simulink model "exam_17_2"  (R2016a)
settings: Solver=ode15s  StartTime=0.0  StopTime=0.2  RelTol=1e-3
libraries: powerlib x9

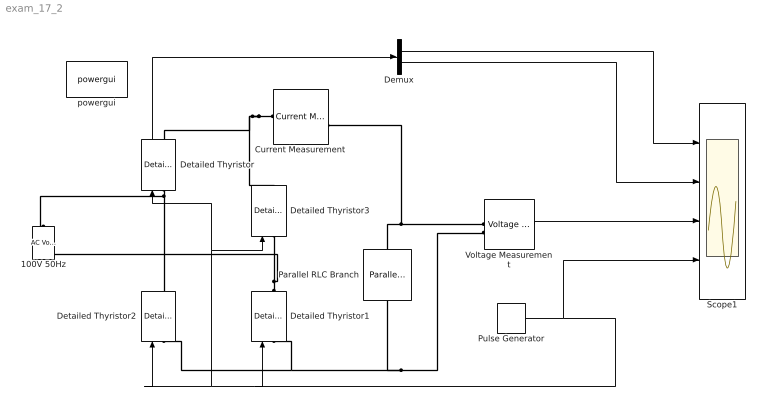
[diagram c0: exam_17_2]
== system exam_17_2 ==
  100V 50Hz : powerlib/Electrical Sources/AC Voltage Source  Amplitude=100  Phase=0  Frequency=50  SampleTime=0  Measurements=None  BusType=swing  Pref=10e3  Qref=0  Qmin=-inf  Qmax=+inf
  Current Measurement : powerlib/Measurements/Current Measurement  PhasorSimulation=off  OutputType=Complex  PSBequivalent=0
  Demux : Demux  Outputs=2
  Detailed Thyristor{,1..3} (4 alike) : powerlib/Power Electronics/Detailed Thyristor  Ron=0.001  Lon=1e-3  Vf=0.8  IL=0.1  Tq=100e-6  IC=0  Rs=500  Cs=250e-9  Measurements=on
  Parallel RLC Branch : powerlib/Elements/Parallel RLC Branch  LConnTagsString=a  RConnTagsString=__new0  BranchType=R  Resistance=1  Inductance=1e-3  SetiL0=off  InitialCurrent=0  Capacitance=1e-6  Setx0=off  InitialVoltage=0  Measurements=None
  Pulse Generator : DiscretePulseGenerator  PulseType=Time based  Period=0.01  PulseWidth=50  PhaseDelay=0.0017
  Scope1 : Scope  NumInputPorts=4
  Voltage Measurement : powerlib/Measurements/Voltage Measurement  PhasorSimulation=off  OutputType=Complex  PSBequivalent=0
  powergui : powerlib/powergui  Priority=1  SimulationMode=Continuous  SolverType=Tustin/Backward Euler (TBE)  SampleTime=50e-6  frequency=60  SPID=off  DisableSnubberDevices=off  DisableRonSwitches=off  DisableVfSwitches=off  SwTol=0  DisplayEquations=off  Interpol=off  ExternalGateDelay=off  methode=off  Ts=10  FunctionMessages=off  echomessages=off  HookPort=off  EnableUseOfTLC=off  x0status=blocks  frequencyindice=50  Pbase=100e6  ErrMax=1e-4  Iterations=50  UnitsV=kV  UnitsW=MW  buscounter=0  RestoreLinks=warning  ResistiveCurrentMeasurement=off  Frange=[0:2:500]  Ylog=off  Xlog=on  ShowGrid=off  save=off  variable=ZData  structure=0  ZoomFFT=off  StartTime=0.0  cycles=1  DisplayStyle=1  fundamental=60  FreqAxis=off  MaxFrequency=1000  frequencyindicesteady=1  RmsSteady=1  display=off
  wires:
  Detailed Thyristor/1 -> Demux/1
  Pulse Generator/1 -> Scope1/4, Detailed Thyristor2/1, Detailed Thyristor3/1, Detailed Thyristor/1, Detailed Thyristor1/1
  Demux/1 -> Scope1/1
  Demux/2 -> Scope1/2
  Voltage Measurement/1 -> Scope1/3
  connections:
  Detailed Thyristor/LConn1 -- Detailed Thyristor2/RConn1 -- 100V 50Hz/RConn1
  Current Measurement/LConn1 -- Detailed Thyristor/RConn1 -- Detailed Thyristor3/RConn1
  Voltage Measurement/LConn1 -- Parallel RLC Branch/LConn1 -- Current Measurement/RConn1
  Voltage Measurement/LConn2 -- Parallel RLC Branch/RConn1 -- Detailed Thyristor2/LConn1 -- Detailed Thyristor1/LConn1
  Detailed Thyristor1/RConn1 -- 100V 50Hz/LConn1 -- Detailed Thyristor3/LConn1
